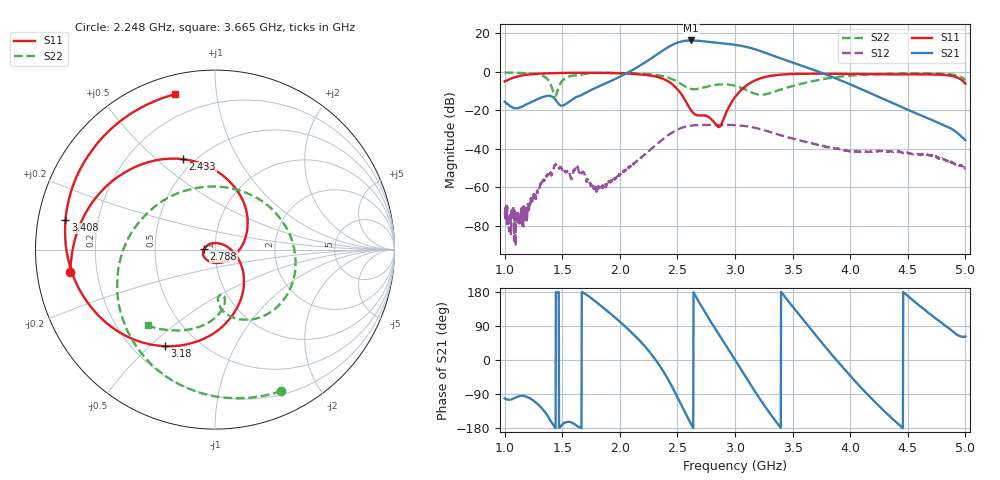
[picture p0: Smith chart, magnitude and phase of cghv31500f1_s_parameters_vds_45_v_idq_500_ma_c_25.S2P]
!Keysight Technologies,E5071C,MY46632031,B.14.03
!Date: Fri Jul 09 16:06:30 2021
!Data & Calibration Information:
!Freq	S11:SOLT2(ON)	S21:SOLT2(ON)	S12:SOLT2(ON)	S22:SOLT2(ON)
!PortZ  Port1:50+j0  Port2:50+j0
!Above PortZ is port z conversion or system Z0 setting when saving the data.
!When reading, reference impedance value at option line is always used.
# Hz S dB R 50
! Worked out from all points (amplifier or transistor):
!   1601 points, 1 GHz to 5 GHz, reference 50 ohm
!   highest |S21| = 16.3 dB at 2.62 GHz (marker M1)
!   |S21| within 3 dB of that: 2.433 GHz to 3.07 GHz (637 MHz wide, 23.1 % of centre)
!   unconditionally stable (mu >= 1): start of sweep to end of sweep
!   at 1.665 GHz: K = 26.66, MAG = 3.0 dB, |S12| = -52.7 dB
!   at 3 GHz: K = 1.89, MAG = 15.5 dB, |S12| = -27.7 dB
!   at 5 GHz: K = 4609.67, MAG = -32.4 dB, |S12| = -50.1 dB
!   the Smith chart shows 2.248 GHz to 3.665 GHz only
!   S11 on the Smith chart (normalised r, x): 2.248 GHz: 0.10, -0.08; 2.433 GHz: 0.44, +0.61; 2.788 GHz: 0.89, +0.01; 3.18 GHz: 0.33, -0.56; 3.408 GHz: 0.08, +0.10; 3.665 GHz: 0.09, +0.77
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1e9  -5.01 154.1  -15.48 -101.3  -72.78 136.7  -0.38 122.4
1.315e9  -0.90 75.4  -13.47 -124.6  -57.73 -131.0  -1.70 61.5
1.6675e9  -0.49 -15.3  -12.08 -180.0  -52.86 -163.3  -1.45 54.8
2.0225e9  -0.78 -104.4  -1.88 95.1  -52.68 10.9  -0.66 -14.1
2.2475e9  -1.77 -171.0  5.99 25.4  -41.45 -56.6  -1.21 -64.9
2.335e9  -2.83 155.8  9.54 -9.9  -37.00 -94.0  -1.80 -91.8
2.4325e9  -5.44 109.5  13.28 -58.4  -32.47 -142.4  -3.28 -131.7
2.525e9  -10.90 53.0  15.65 -113.1  -29.43 162.7  -6.09 175.6
2.62e9  -20.15 -32.1  16.31 -169.8  -28.00 106.2  -8.93 105.3
2.71e9  -22.69 -130.3  15.98 141.1  -27.66 57.0  -8.45 44.1
2.7875e9  -24.30 176.1  15.48 102.2  -27.65 18.3  -7.28 6.6
2.905e9  -23.80 18.2  14.72 46.1  -27.67 -37.4  -6.49 -36.1
3e9  -13.17 -43.1  14.03 0.6  -27.74 -82.8  -7.25 -64.1
3.095e9  -7.35 -84.1  13.00 -45.5  -28.29 -128.0  -9.37 -83.2
3.18e9  -4.34 -117.6  11.62 -86.1  -29.24 -168.5  -11.52 -86.2
3.2875e9  -2.37 -155.3  9.38 -134.1  -31.01 143.3  -11.39 -78.8
3.4075e9  -1.42 168.9  6.77 176.9  -33.11 94.7  -9.01 -85.8
3.665e9  -0.98 104.6  1.36 78.5  -37.13 -1.2  -4.97 -131.5
3.6675e9  -0.97 104.1  1.31 77.6  -37.29 -2.1  -4.93 -132.1
4.335e9  -1.30 -65.3  -15.39 -146.2  -41.38 177.3  -0.99 62.7
4.7e9  -1.35 -165.3  -24.84 119.4  -43.59 89.8  -0.81 -0.6
5e9  -6.24 120.2  -35.60 62.2  -50.14 35.6  -4.26 -50.0
